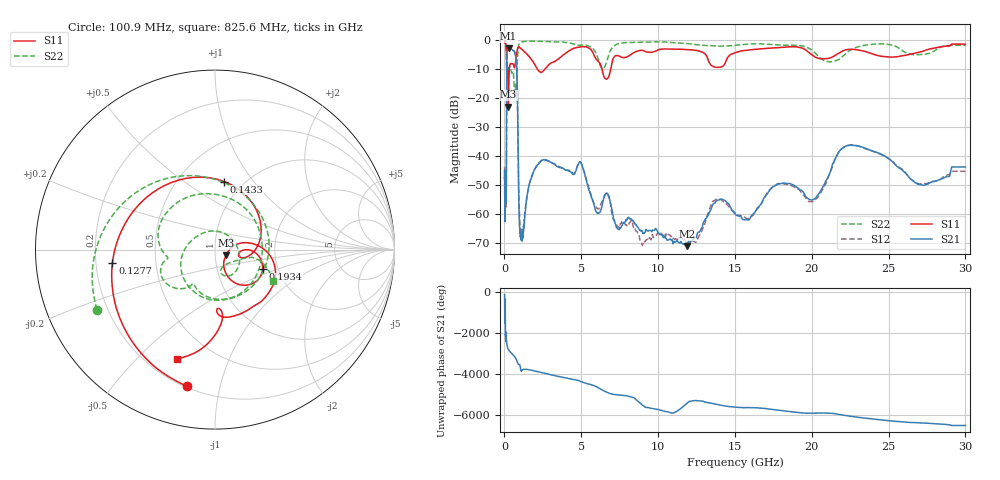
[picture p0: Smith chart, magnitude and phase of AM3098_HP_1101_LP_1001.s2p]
! Date/Time: Thu, Feb 28, 2019 8:45 AM
! Network Analyzer: Agilent Technologies E8364B Rev: A.07.50.67
! Sweep from 0.010 to 30.000 GHz, 1601 Points, Sweep Type: LOG
! Power Supply: 5.022 V, 0.002 A
# Hz S DB R 50
!freq MagS11 AngS11 MagS21 AngS21 MagS12 AngS12 MagS22 AngS22
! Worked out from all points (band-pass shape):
!   1601 points, 10 MHz to 30 GHz, reference 50 ohm
!   highest |S21| = -3.07 dB at 266.5 MHz (marker M1); lowest = -71.2 dB at 11.89 GHz (marker M2)
!   |S21| within 3 dB of the highest: 159.3 MHz to 736.2 MHz (576.9 MHz wide, 129 % of centre)
!   lowest |S11| = -23.1 dB at 252.2 MHz (marker M3), VSWR 1.15, Z = 56.5 - j3.55 ohm
!   |S11| at or under -10 dB: 147.9 MHz to 320.5 MHz (172.6 MHz wide, 73.7 % of centre); 2.119 GHz to 2.665 GHz (546.3 MHz wide, 22.8 % of centre); 6.342 GHz to 6.923 GHz (581.5 MHz wide, 8.77 % of centre)
!   |S22| runs from -19.8 to -0.5 dB; largest |S21 - S12| = 0.0097
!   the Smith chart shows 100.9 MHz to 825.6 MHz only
!   S11 on the Smith chart (normalised r, x): 100.9 MHz: 0.21, -0.79; 127.7 MHz: 0.27, -0.06; 143.3 MHz: 0.82, +0.73; 193.4 MHz: 1.66, -0.39; 825.6 MHz: 0.32, -0.66
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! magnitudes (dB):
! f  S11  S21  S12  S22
! 10 MHz  -0.4  -47.9  -43.9  -0.6
! 38.04 MHz  -0.3  -57.6  -59.6  -0.8
! 100.9 MHz  -2.2  -53.3  -53.9  -2.6
! 127.7 MHz  -4.8  -41.3  -40.9  -6.2
! 143.3 MHz  -8.3  -15.9  -15.9  -10.5
! 144.7 MHz  -8.8  -14.3  -14.2  -10.6
! 193.4 MHz  -10.9  -3.9  -3.9  -9.7
! 252.2 MHz  -23.1  -3.1  -3.1  -11.5
! 266.5 MHz  -19.4  -3.1  -3.0  -11.4
! 550.5 MHz  -8.3  -3.8  -3.7  -10.9
! 669.1 MHz  -9.5  -4.4  -4.3  -19.7
! 825.6 MHz  -3.8  -14.6  -14.5  -8.7
! 949.8 MHz  -2.5  -59.1  -56.7  -1.5
! 1.044 GHz  -3.0  -68.1  -66.9  -1.0
! 2.084 GHz  -9.6  -43.8  -43.5  -0.6
! 4.927 GHz  -2.5  -42.1  -42.2  -1.9
! 7.926 GHz  -6.1  -62.0  -63.8  -1.0
! 11.89 GHz  -3.4  -71.2  -69.0  -1.4
! 13.95 GHz  -9.6  -55.3  -54.9  -2.2
! 20.1 GHz  -5.6  -55.1  -55.7  -4.0
! 22.56 GHz  -3.4  -36.4  -36.3  -3.5
! 30 GHz  -1.6  -43.9  -45.4  -2.0
